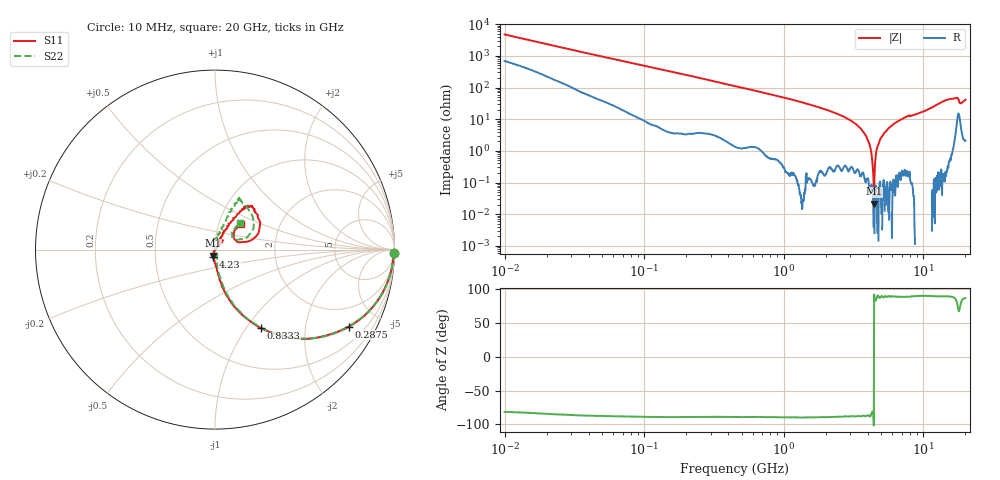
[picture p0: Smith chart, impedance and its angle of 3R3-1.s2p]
!Keysight Technologies,P5008B,MY61100088,A.16.20.02
!Date: Monday, May 27, 2024 14:53:23
!Correction: S11(C* 2-Port  )
!S21(C* 2-Port  )
!S12(C* 2-Port  )
!S22(C* 2-Port  )
!S2P File: Measurements: S11, S21, S12, S22:Log Frequency Sweep
# Hz S  dB  R 50
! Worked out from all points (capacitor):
!   1601 points, 10 MHz to 20 GHz, reference 50 ohm
!   read as one part in series: C = 3.42 pF near 10.39 MHz
!   lowest |Z| = 21.5 mohm at 4.436 GHz (marker M1)
!   series resonance near 4.43 GHz, so ESL is about 380 pH
!   S11 on the Smith chart (normalised r, x): 10 MHz: 5, -95; 287.5 MHz: 1.05, -3.44; 833.3 MHz: 1.00, -1.17; 4.23 GHz: 0.98, -0.08; 20 GHz: 1.27, +0.38
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1e7  -0.01 -1.2  -33.51 80.5  -33.50 80.5  -0.03 -1.2
3.555162e7  -0.06 -4.2  -22.49 82.7  -22.50 82.7  -0.06 -4.3
1.263918e8  -0.32 -14.5  -12.10 74.7  -12.12 74.7  -0.31 -14.5
2.875032e8  -1.31 -29.9  -6.09 58.9  -6.10 59.0  -1.32 -29.9
4.472136e8  -2.65 -42.0  -3.55 47.4  -3.55 47.4  -2.63 -41.9
8.332721e8  -5.90 -59.7  -1.34 30.0  -1.35 30.0  -5.89 -59.3
1.589917e9  -11.32 -75.2  -0.33 15.0  -0.34 15.0  -11.27 -74.1
2.962417e9  -18.95 -84.0  -0.05 4.4  -0.06 4.4  -18.98 -81.7
4.230405e9  -27.60 -104.2  0.00 -1.1  -0.01 -1.1  -28.48 -70.0
4.436224e9  -28.83 -109.5  0.00 -1.9  -0.01 -1.9  -29.81 -70.8
4.924959e9  -36.49 -118.5  0.01 -3.5  0.00 -3.5  -35.77 -52.9
5.339198e9  -47.53 -139.6  0.01 -4.7  0.00 -4.7  -46.25 -39.0
5.493573e9  -48.20 17.3  0.02 -5.2  0.01 -5.2  -48.81 9.1
5.652411e9  -43.08 68.5  0.02 -5.6  0.00 -5.6  -44.17 82.4
5.983999e9  -35.47 56.7  0.02 -6.6  0.01 -6.6  -36.73 95.8
6.275133e9  -31.57 54.9  0.02 -7.4  0.01 -7.4  -32.71 99.6
7.624508e9  -24.27 49.1  0.01 -10.9  0.00 -10.9  -25.05 96.2
9.577292e9  -24.86 62.7  0.03 -15.5  0.02 -15.5  -24.61 83.9
1.503978e10  -10.28 53.1  -0.38 -29.4  -0.39 -29.4  -10.30 65.0
1.717946e10  -10.27 38.7  -0.75 -34.5  -0.75 -34.5  -10.57 52.8
1.871311e10  -18.18 32.0  -0.40 -30.9  -0.41 -30.9  -18.38 38.4
2e10  -13.88 44.6  -0.30 -36.7  -0.31 -36.8  -13.76 47.2
